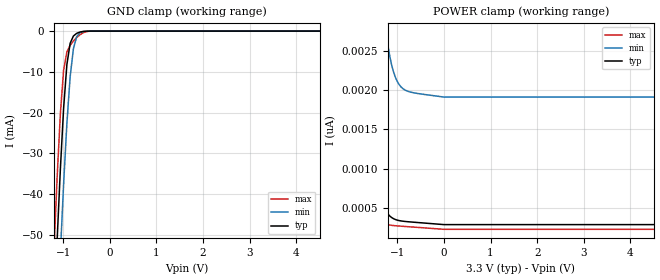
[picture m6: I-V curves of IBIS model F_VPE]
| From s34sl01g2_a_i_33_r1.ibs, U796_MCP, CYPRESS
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|   Model   F_VPE
[Model]   F_VPE
Model_type Input
Vinl =   0.6600V
Vinh =   2.6400V
   C_comp   2.0094pF   2.0040pF   2.0107pF
[Temperature Range]   25.0000   0.1050k   -40.0000
[Pullup Reference]   3.3000V   3.0000V   3.6000V
[Pulldown Reference]   0.0V   0.0V   0.0V
[POWER Clamp Reference]   3.3000V   3.0000V   3.6000V
[GND Clamp Reference]   0.0V   0.0V   0.0V
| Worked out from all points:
|   GND clamp passes 1 mA (typ) near -0.76 V on its own axis
[GND_clamp]
|Voltage   I(typ)   I(min)   I(max)
-3.3V     -739.7mA   -757.8mA   -727.1mA
-1.2V     -70.6mA    -92.49mA   -54.59mA
-1.13V    -51.52mA   -73.07mA   -36.13mA
-1.06V    -33.94mA   -54.59mA   -20.29mA
-990mV    -18.9mA    -37.51mA   -9.564mA
-920mV    -8.215mA   -22.66mA   -5.118mA
-850mV    -2.991mA   -11.22mA   -3.486mA
-780mV    -1.209mA   -4.318mA   -2.439mA
-710mV    -553.4uA   -1.357mA   -1.585mA
-570mV    -84.76uA   -121uA     -415.6uA
-360mV    -1.285uA   -5.784uA   -4.845uA
6.6V      287.4pA    1.936nA    214.2pA
[POWER_clamp]
|Voltage   I(typ)   I(min)   I(max)
-3.28V    2.645uA    1.278uA    5.729uA
-1.84V    8.137nA    23.44nA    3.41nA
-1.8V     6.404nA    19.46nA    2.663nA
-1.76V    5.038nA    16.2nA     2.089nA
-1.68V    3.13nA     11.33nA    1.31nA
-1.64V    2.478nA    9.544nA    1.051nA
-1.56V    1.581nA    6.896nA    702.2pA
-1.48V    1.05nA     5.144nA    502pA
-1.24V    455.2pA    2.745nA    297pA
-1V       344pA      2.111nA    270.6pA
-640mV    317.4pA    1.966nA    254.8pA
6.6V      287.1pA    1.912nA    227.2pA
